[IBIS Ver]   3.2
[File name]   sprm349a.ibs
[File Rev]   1.0
[Date]   Monday Aug 10  2009
[Source]   IBIS Model Generated from PACED 4.51D
[Notes]
|   Technology type SR50
|   Warnings such as non-montonic behavior at the noisy end
|   points of the slopes or TVCurves not asymptotically
|   approaching a final value can be ignored.
[Disclaimer]   Please be aware that in the absence of a written agreement
|   Texas Instruments(TI) assumes no liability for:
|   (1) The accuracy of the IBIS models provided to your company
|   (2) The proper functioning of these Models in your design
|   or for any resulting applications;or
|   property rights resulting from your use of these models.
|   This information is for modeling purposes only
|   and is not guaranteed.
|   TI provides IBIS Models as a service to our customers and
|   therefore reserves the right to limit distribution of the
|   Models.
[Copyright]   Property of Texas Instruments Incorporated.
|   Unauthorised reproduction and/or distribution is strictly.
|   prohibited.
|   This product is protected under copyright law and trade
|   secret law as an unpublished work.
|   Created 1999,(C) Copyright 1999-2001,
|   Texas Instruments Incorporated., All Rights Reserved.
[Component]   C6452   | 529 pin
[Manufacturer]   Texas Instruments
[Package]
| Variable   Typ   Min   Max
R_pkg   0.0   0.0   0.0
L_pkg   0.0   0.0   0.0
C_pkg   0.0   0.0   0.0
[Pin]   signal_name   model_name   R_pin   L_pin   C_pin
M1   CLKIN1   THYPDFZP18   1.03E+00   2.43E-09   1.57E-12
F1   CLKIN2   THYPDFZP18   1.24E+00   3.00E-09   1.65E-12
M3   SYSCLK4   EPUFZSCP18   6.07E-01   2.05E-09   1.32E-12
| JTAG
H23   TCLK   KP18PUSR50   1.14E+00   2.78E-09   1.62E-12
J22   TDI   THYPUFZP18   1.10E+00   2.58E-09   1.66E-12
J23   TDO   EPUFZSCP18   1.16E+00   2.67E-09   1.47E-12
L22   TMS   THYPUFZP18   9.03E-01   2.34E-09   1.52E-12
L23   TRSTz   THYPDFZP18   1.03E+00   2.62E-09   1.41E-12
K23   EMU0   EPUFZSCP18   1.08E+00   2.62E-09   1.49E-12
K22   EMU1   EPUFZSCP18   1.02E+00   2.47E-09   1.58E-12
K21   EMU2   EPUFZSCP18   7.51E-01   2.07E-09   1.39E-12
K20   EMU3   EPUFZSCP18   5.34E-01   1.66E-09   1.26E-12
L18   EMU4   EPUFZSCP18   2.72E-01   1.21E-09   1.07E-12
J21   EMU5   EPUFZSCP18   8.00E-01   2.22E-09   1.48E-12
K19   EMU6   EPUFZSCP18   4.11E-01   1.49E-09   1.19E-12
H21   EMU7   EPUFZSCP18   9.35E-01   2.47E-09   1.51E-12
J20   EMU8   EPUFZSCP18   6.07E-01   1.77E-09   1.33E-12
H20   EMU9   EPUFZSCP18   6.51E-01   1.98E-09   1.35E-12
J19   EMU10   EPUFZSCP18   4.39E-01   1.54E-09   1.18E-12
K18   EMU11   EPUFZSCP18   1.61E-01   1.32E-09   9.70E-13
| Reset/Interrupts
J18   NMI   SHYPDFZP18   1.68E-01   9.30E-10  9.90E-13
H19   RESETSTATz   CSHYPUFZP18   4.23E-01   1.44E-09  1.19E-12
G20   RESETz   IT33SHYP18   7.57E-01   2.04E-09  1.41E-12
|HOST-PORT INTERFACE (HPI) or PCI
AA22   AD00/HD00   CGPDFZP18   1.13E+00   3.06E-09  1.65E-12
AB22   AD01/HD01   CGPDFZP18   1.30E+00   2.94E-09  1.77E-12
AC21   AD02/HD02   CGPDFZP18   1.43E+00   3.03E-09  1.82E-12
AA23   AD03/HD03   CGPDFZP18   1.33E+00   3.36E-09  1.62E-12
AC22   AD04/HD04   CGPDFZP18   1.48E+00   3.26E-09  1.78E-12
AB21   AD05/HD05   CGPDFZP18   1.20E+00   2.86E-09  1.78E-12
AA21   AD06/HD06   CGPDFZP18   1.21E+00   2.84E-09  1.75E-12
Y21   AD07/HD07   CGPDFZP18   9.64E-01   2.45E-09  1.56E-12
AB20   AD08/HD08   CGPDFZP18   1.32E+00   3.07E-09  1.77E-12
AA20   AD09/HD09   CGPDFZP18   1.12E+00   2.60E-09  1.71E-12
Y20   AD10/HD10   CGPDFZP18   9.03E-01   2.30E-09  1.53E-12
Y19   AD11/HD11   CGPDFZP18   7.65E-01   2.00E-09  1.46E-12
AB18   AD12/HD12   CGPDFZP18   1.03E+00   2.44E-09  1.57E-12
AA19   AD13/HD13   CGPDFZP18   9.67E-01   2.55E-09  1.60E-12
AC18   AD14/HD14   CGPDFZP18   1.25E+00   2.84E-09  1.66E-12
AA18   AD15/HD15   CGPDFZP18   9.00E-01   2.41E-09  1.56E-12
Y16   AD16/HD16   CGPDFZP18   5.39E-01   1.78E-09  1.28E-12
AB15   AD17/HD17   CGPDFZP18   8.91E-01   2.20E-09  1.44E-12
AA15   AD18/HD18   CGPDFZP18   6.70E-01   1.96E-09  1.40E-12
Y15   AD19/HD19   CGPDFZP18   5.61E-01   1.77E-09  1.30E-12
W15   AD20/HD20   CGPDFZP18   3.46E-01   1.54E-09  1.13E-12
V15   AD21/HD21   CGPDFZP18   3.24E-01   1.93E-09  1.13E-12
AC14   AD22/HD22   CGPDFZP18   9.71E-01   2.39E-09  1.40E-12
AB14   AD23/HD23   CGPDFZP18   8.86E-01   2.29E-09  1.52E-12
W14   AD24/HD24   CGPDFZP18   2.58E-01   1.37E-09  1.09E-12
V14   AD25/HD25   CGPDFZP18   2.33E-01   1.28E-09  1.03E-12
AC13   AD26/HD26   CGPDFZP18   9.46E-01   2.52E-09  1.41E-12
AB13   AD27/HD27   CGPDFZP18   7.59E-01   2.10E-09  1.23E-12
AA13   AD28/HD28   CGPDFZP18   6.92E-01   2.01E-09  1.37E-12
Y13   AD29/HD29   CGPDFZP18   4.89E-01   1.66E-09  1.24E-12
W13   AD30/HD30   CGPDFZP18   3.65E-01   1.49E-09  1.13E-12
V13   AD31/HD31   CGPDFZP18   1.74E-01   1.14E-09  9.80E-13
W19   PPAR/HASz   CGPUFZP18   7.38E-01   2.23E-09  1.44E-12
Y18   PSTOPz/HCNTL0   CGPDFZP18   7.33E-01   2.05E-09  1.38E-12
Y17   PDEVSELz/HCNTL1   CGPDFZP18   6.59E-01   1.94E-09  1.35E-12
W17   PPERRz/HCSz   CGPUFZP18   5.02E-01   1.71E-09  1.25E-12
W18   PSERRz/HDS1z   CGPUFZP18   5.99E-01   1.94E-09  1.34E-12
AC17   PCBE1z/HDS2z   CGPUFZP18   1.37E+00   3.05E-09  1.74E-12
W16   PCBE2z/HRWz   CGPUFZP18   3.90E-01   1.62E-09  1.18E-12
AC15   PCLK/HHWIL   CGPUFZP18   1.21E+00   2.83E-09  1.65E-12
AA16   PFRAMEz/HINTz   CGPUFZP18   8.21E-01   2.15E-09  1.48E-12
AB17   PIRDYz/HRDYz   CGPUFZP18   8.74E-01   2.33E-09  1.51E-12
U13   PGNTz/GP00   CGPDFZP18   8.20E-02   6.60E-10  9.90E-13
U12   PRSTz/GP01   CGPDFZP18   1.95E-01   1.77E-09  9.90E-13
V12   PINTAz/GP02   CGPDFZP18   1.12E-01   7.50E-10  9.30E-13
AA12   PREQz/GP03   CGPDFZP18   6.04E-01   2.11E-09  1.30E-12
AC20   PCBE0z/GP04   CGPDFZP18   1.50E+00   3.44E-09  1.79E-12
AA17   PTRDYz/GP05   CGPDFZP18   7.78E-01   2.20E-09  1.44E-12
AA14   PIDSEL/GP06   CGPDFZP18   7.10E-01   2.03E-09  1.31E-12
Y14   PCBE3z/GP07   CGPDFZP18   5.13E-01   1.76E-09  1.26E-12
| CONFIGURATION AND EMIFA
F2   DEVICEENABLE0/AEA20 PDFZSCP18   1.10E-03   2.71E-09  1.69E-12
G3   EMIFAWIDTH/AEA22   PDFZSCP18   9.26E-01   2.45E-09  1.55E-12
G2   FASTBOOT/AEA21   PDFZSCP18   9.83E-01   2.39E-09  1.49E-12
H2   UHPIEN   THYPDFZP18   9.16E-01   2.19E-09  1.46E-12
H3   HPIWIDTH/AEA16   PDFZSCP18   6.86E-01   1.84E-09  1.39E-12
H6   RSVBOOT/AEA15   DPUFZSCP18   3.83E-01   1.80E-09  1.17E-12
G5   PCI66/AEA18   PDFZSCP18   6.50E-01   1.95E-09  1.43E-12
F3   BOOTMODE0/AEA11   PDFZSCP18   9.09E-01   2.46E-09  1.57E-12
F4   BOOTMODE1/AEA12   PDFZSCP18   8.43E-01   2.38E-09  1.53E-12
F5   BOOTMODE2/AEA13   PDFZSCP18   7.20E-01   2.13E-09  1.45E-12
G6   BOOTMODE3/AEA14   PDFZSCP18   4.32E-01   1.86E-09  1.30E-12
|I2C
D22   SCL0   BI2CSFZP18   1.07E+00   2.64E-09  1.65E-12
C23   SDA0   BI2CSFZP18   1.34E+00   3.18E-09  1.72E-12
| MDIO
U9   MDCLK   BTHYPDFZP18   4.31E-02   1.01E-09  8.90E-13
U8   MDIO   BTHYPUFZP18   3.15E-01   1.51E-09  1.08E-12
| SPI or UART
F22   SPICLK   CSHYPUFZP18   9.92E-01   2.41E-09  1.5E-12
D23   SPICS1z/UARTTX   CSHYPUFZP18   1.17E+00   2.88E-09  1.63E-12
F23   SPICS2z/UARTRX   CSHYPUFZP18   1.11E+00   2.71E-09  1.47E-12
G23   SPIDI/UARTRTS   CSHYPUFZP18   1.09E+00   2.68E-09  1.36E-12
F21   SPIDO/UARTCTS   CSHYPUFZP18   8.04E-01   2.27E-09  1.48E-12
| TIMER 0/1 or GPIO[8:11]
E20   T0INP12/GP08   CSHYPDFZP18   6.60E-01   1.98E-09  1.36E-12
D21   T0OUT12/GP09   CSHYPDFZP18   8.34E-01   2.18E-09  1.52E-12
E21   T1INP12/GP10   CSHYPDFZP18   7.81E-01   2.11E-09  1.47E-12
C22   T1OUT12/GP11   CSHYPDFZP18   1.13E+00   2.53E-09  1.64E-12
| MCASP
AC4   AHCLKR_TSIP1CLKA   HYPDFZP18   1.27E+00   3.13E-09  1.70E-12
AC3   AHCLKX_TSIP1CLKB   HYPDFZP18   1.37E+00   3.11E-09  1.76E-12
AC6   ACLKR_TSIP0CLKA   PDFZSCP18   1.22E+00   3.03E-09  1.58E-12
AC7   ACLKX_TSIP0CLKB   PDFZSCP18   1.06E+00   2.81E-09  1.59E-12
W6   AFSR_TSIP0FSA   HYPDFZP18   4.85E-01   1.75E-09  1.24E-12
AA7   AFSX_TSIP0FSB   HYPDFZP18   7.10E-01   2.09E-09  1.40E-12
AB6   AXR0_TSIP0TR0   HYPDFZP18   9.44E-01   2.37E-09  1.54E-12
Y6   AXR1_TSIP0TR1   HYPDFZP18   6.21E-01   2.01E-09  1.34E-12
AA6   AXR2_TSIP0TX0   HYPDFZP18   9.61E-01   2.55E-09  1.57E-12
AB4   AXR3_TSIP0TX1   HYPDFZP18   1.10E+00   2.75E-09  1.69E-12
Y5   AXR4_TSIP1TR0   HYPDFZP18   7.78E-01   2.33E-09  1.45E-12
V7   AXR5_TSIP1TR1   HYPDFZP18   2.85E-01   1.44E-09  1.09E-12
AA4   AXR6_TSIP1TX0   HYPDFZP18   8.69E-01   2.37E-09  1.53E-12
V6   AXR7_TSIP1TX1   HYPDFZP18   3.46E-01   1.47E-09  1.11E-12
Y7   AXR8   HYPDFZP18   5.14E-01   1.78E-09  1.26E-12
AA5   AXR9   HYPDFZP18   8.91E-01   2.30E-09  1.53E-12
AB3   AMUTEIN_TSIP1FSA   HYPDFZP18   1.08E+00   2.69E-09  1.62E-12
U7   AMUTE_TSIP1FSB   HYPDFZP18   9.10E-02   1.07E-09  9.00E-13
|GPIO[12:15]
V21   GP12   PDFZSCP18   7.68E-01   2.09E-09  1.39E-12
T19   GP13   PDFZSCP18   2.80E-01   1.46E-09  1.09E-12
T20   GP14   PDFZSCP18   5.40E-01   1.81E-09  1.29E-12
T21   GP15   PDFZSCP18   6.41E-01   1.96E-09  1.34E-12
|GPIO[16:31]
R19   GP16   PDFZSCP18   3.50E-01   1.59E-09  1.12E-12
P19   GP17   PDFZSCP18   2.74E-01   1.37E-09  1.08E-12
P18   GP18   PDFZSCP18   5.46E-02   8.00E-10  9.20E-13
R22   GP19   PDFZSCP18   7.90E-01   2.27E-09  1.39E-12
R21   GP20   PDFZSCP18   6.22E-01   1.90E-09  1.18E-12
R20   GP21   PDFZSCP18   4.22E-01   1.59E-09  1.19E-12
N21   GP22   PDFZSCP18   6.84E-01   1.87E-09  1.34E-12
N20   GP23   PDFZSCP18   4.77E-01   1.60E-09  1.23E-12
N19   GP24   PDFZSCP18   3.36E-01   1.45E-09  1.12E-12
P21   GP25   PDFZSCP18   6.15E-01   1.78E-09  1.32E-12
P20   GP26   PDFZSCP18   4.98E-01   1.67E-09  1.23E-12
M20   GP27   PDFZSCP18   4.31E-01   1.55E-09  1.20E-12
M18   GP28   PDFZSCP18   2.42E-01   9.50E-10  1.05E-12
N18   GP29   PDFZSCP18   1.11E-01   1.36E-09  9.30E-13
M21   GP30   PDFZSCP18   6.50E-01   1.91E-09  1.37E-12
M19   GP31   PDFZSCP18   3.69E-01   1.50E-09  1.16E-12
|VLYNQ
W1   VCLK   EPUFZSCP18   1.37E+00   2.98E-09  1.82E-12
Y1   VSCRUNz   DPUFZSCP18   1.21E+00   2.87E-09  1.56E-12
W2   VRXD0   PDFZSCP18   1.04E+00   2.57E-09  1.57E-12
V3   VRXD1   PDFZSCP18   7.50E-01   2.13E-09  1.43E-12
V4   VRXD2   PDFZSCP18   6.91E-01   1.93E-09  1.37E-12
U1   VRXD3   PDFZSCP18   1.11E+00   2.71E-09  1.39E-12
U3   VTXD0   PDFZSCP18   6.30E-01   2.07E-09  1.36E-12
U2   VTXD1   PDFZSCP18   9.93E-01   2.48E-09  1.55E-12
U5   VTXD2   PDFZSCP18   4.26E-01   1.65E-09  1.18E-12
U4   VTXD3   PDFZSCP18   5.54E-01   1.83E-09  1.28E-12
|EMIFA
T1   AECLKIN   PDFZSCP18   1.10E+00   2.68E-09  1.57E-12
P1   AECLKOUT   ETHYPDFZSCP18   1.29E+00   3.05E-09  1.58E-12
T2   ASDWEz   DPUFZSCP18   9.53E-01   2.50E-09  1.48E-12
R1   ARNW   DPUFZSCP18   1.16E+00   2.90E-09  1.56E-12
P2   AOE   DPUFZSCP18   1.35E+00   3.01E-09  1.88E-12
T6   AED00   DPUFZSCP18   4.61E-01   1.80E-09  1.23E-12
T5   AED01   DPUFZSCP18   4.48E-01   1.70E-09  1.20E-12
T4   AED02   DPUFZSCP18   5.57E-01   1.94E-09  1.29E-12
T3   AED03   DPUFZSCP18   6.26E-01   2.10E-09  1.36E-12
R6   AED04   DPUFZSCP18   2.37E-01   1.30E-09  1.05E-12
R5   AED05   DPUFZSCP18   3.55E-01   1.68E-09  1.13E-12
R4   AED06   DPUFZSCP18   6.30E-01   1.99E-09  1.34E-12
R3   AED07   DPUFZSCP18   7.59E-01   2.16E-09  1.44E-12
R2   AED08   DPUFZSCP18   7.50E-01   2.10E-09  1.47E-12
P6   AED09   DPUFZSCP18   1.95E-01   1.17E-09  1.00E-12
P5   AED10   DPUFZSCP18   2.95E-01   1.57E-09  1.10E-12
P4   AED11   DPUFZSCP18   4.27E-01   1.71E-09  1.19E-12
P3   AED12   DPUFZSCP18   6.58E-01   2.05E-09  1.39E-12
N4   AED13   DPUFZSCP18   4.47E-01   1.74E-09  1.20E-12
N6   AED14   DPUFZSCP18   1.75E-01   1.02E-09  9.60E-13
N5   AED15   DPUFZSCP18   2.68E-01   1.44E-09  1.05E-12
|EMIFA
L1   AARDY   DPUFZSCP18   1.28E+00   3.17E-09  1.67E-12
J2   ABA0   PDFZSCP18   1.04E+00   2.46E-09  1.59E-12
J1   ABA1   PDFZSCP18   1.45E+00   3.33E-09  1.81E-12
K2   AADS   PDFZSCP18   1.04E+00   2.68E-09  1.62E-12
L2   ABE00z   DPUFZSCP18   8.08E-01   2.14E-09  1.47E-12
M4   ABE01z   DPUFZSCP18   4.85E-01   2.09E-09  1.24E-12
M5   AEA10   DPUFZSCP18   2.77E-01   1.46E-09  1.10E-12
L3   ACE2z   DPUFZSCP18   6.73E-01   2.12E-09  1.37E-12
L4   ACE3z   DPUFZSCP18   4.76E-01   1.85E-09  1.21E-12
L5   AEA00   PDFZSCP18   3.66E-01   1.74E-09  1.15E-12
K3   AEA01   PDFZSCP18   8.15E-01   2.25E-09  1.44E-12
K4   AEA02   PDFZSCP18   5.73E-01   1.83E-09  1.30E-12
L6   AEA03   PDFZSCP18   2.93E-01   1.53E-09  1.11E-12
K5   AEA04   PDFZSCP18   4.35E-01   1.59E-09  1.22E-12
J3   AEA05   PDFZSCP18   7.12E-01   2.06E-09  1.42E-12
J4   AEA06   PDFZSCP18   6.99E-01   2.11E-09  1.39E-12
J5   AEA07   PDFZSCP18   5.03E-01   1.86E-09  1.26E-12
J6   AEA08   PDFZSCP18   4.17E-01   1.44E-09  1.22E-12
K6   AEA09   PDFZSCP18   2.68E-01   1.39E-09  1.08E-12
|EMIFA
H4   AEA23   PDFZSCP18   6.03E-01   1.81E-09  1.33E-12
H5   AEA19   DPUFZSCP18   4.13E-01   1.63E-09  1.24E-12
G4   AECLKINSEL/AEA17   PDFZSCP18   7.59E-01   2.14E-09  1.45E-12
|DDR2 Memory Controller
C12   DDR_BA0   BSSTL18GFZ   7.13E-01   2.24E-09  1.37E-12
B12   DDR_BA1   BSSTL18GFZ   9.90E-01   2.87E-09  1.57E-12
E11   DDR_BA2   BSSTL18GFZ   3.69E-01   1.57E-09  1.13E-12
F9   DDR_CSz   BSSTL18GFZ   1.55E-01   9.90E-10  1.00E-12
D15   DDR_A00   BSSTL18GFZ   7.89E-01   2.19E-09  1.45E-12
C15   DDR_A01   BSSTL18GFZ   8.92E-01   2.34E-09  1.53E-12
F13   DDR_A02   BSSTL18GFZ   3.48E-01   1.56E-09  1.20E-12
E14   DDR_A03   BSSTL18GFZ   5.23E-01   1.84E-09  1.29E-12
D14   DDR_A04   BSSTL18GFZ   6.56E-01   2.26E-09  1.35E-12
C14   DDR_A05   BSSTL18GFZ   8.44E-01   2.42E-09  1.49E-12
F11   DDR_A06   BSSTL18GFZ   1.97E-01   1.14E-09  1.00E-12
B14   DDR_A07   BSSTL18GFZ   9.61E-01   2.66E-09  1.45E-12
F12   DDR_A08   BSSTL18GFZ   3.14E-01   1.58E-09  1.16E-12
D13   DDR_A09   BSSTL18GFZ   5.99E-01   2.06E-09  1.32E-12
A13   DDR_A10   BSSTL18GFZ   1.07E+00   2.70E-09  1.58E-12
B13   DDR_A11   BSSTL18GFZ   9.79E-01   2.58E-09  1.50E-12
E12   DDR_A12   BSSTL18GFZ   4.73E-01   1.78E-09  1.22E-12
F10   DDR_A13   BSSTL18GFZ   2.59E-01   1.34E-09  1.11E-12
A12   DDR_CLKN   BSSTL18GFZ   1.07E+00   2.61E-09  1.54E-12
A11   DDR_CLKP   BSSTL18GFZ   1.06E+00   2.52E-09  1.51E-12
E9   DDR_D00   BSSTL18GFZ   2.79E-01   1.37E-09  1.08E-12
C9   DDR_D01   BSSTL18GFZ   7.42E-01   2.03E-09  1.41E-12
B9   DDR_D02   BSSTL18GFZ   8.01E-01   2.33E-09  1.37E-12
C8   DDR_D03   BSSTL18GFZ   6.80E-01   2.06E-09  1.35E-12
E8   DDR_D04   BSSTL18GFZ   2.66E-01   1.23E-09  1.06E-12
D8   DDR_D05   BSSTL18GFZ   5.70E-01   1.82E-09  1.31E-12
C7   DDR_D06   BSSTL18GFZ   6.64E-01   1.96E-09  1.30E-12
E7   DDR_D07   BSSTL18GFZ   3.81E-01   1.51E-09  1.17E-12
C6   DDR_D08   BSSTL18GFZ   7.33E-01   2.12E-09  1.40E-12
B7   DDR_D09   BSSTL18GFZ   8.07E-01   2.19E-09  1.45E-12
D6   DDR_D10   BSSTL18GFZ   6.12E-01   1.98E-09  1.32E-12
A3   DDR_D11   BSSTL18GFZ   1.30E+00   3.23E-09  1.59E-12
B3   DDR_D12   BSSTL18GFZ   1.18E+00   2.81E-09  1.65E-12
A4   DDR_D13   BSSTL18GFZ   1.06E+00   2.72E-09  1.60E-12
B4   DDR_D14   BSSTL18GFZ   9.80E-01   2.53E-09  1.51E-12
C5   DDR_D15   BSSTL18GFZ   7.44E-01   2.27E-09  1.42E-12
B16   DDR_D16   BSSTL18GFZ   1.14E+00   2.74E-09  1.60E-12
C16   DDR_D17   BSSTL18GFZ   1.03E+00   2.67E-09  1.61E-12
D16   DDR_D18   BSSTL18GFZ   8.61E-01   2.33E-09  1.46E-12
E16   DDR_D19   BSSTL18GFZ   7.90E-01   2.29E-09  1.38E-12
B17   DDR_D20   BSSTL18GFZ   1.20E+00   2.84E-09  1.71E-12
C17   DDR_D21   BSSTL18GFZ   1.11E+00   2.73E-09  1.38E-12
D17   DDR_D22   BSSTL18GFZ   9.15E-01   2.28E-09  1.42E-12
E17   DDR_D23   BSSTL18GFZ   8.53E-01   2.19E-09  1.49E-12
C18   DDR_D24   BSSTL18GFZ   1.26E+00   3.10E-09  1.75E-12
D18   DDR_D25   BSSTL18GFZ   1.06E+00   2.53E-09  1.50E-12
B19   DDR_D26   BSSTL18GFZ   1.50E+00   3.33E-09  1.82E-12
C19   DDR_D27   BSSTL18GFZ   1.28E+00   3.03E-09  1.73E-12
B20   DDR_D28   BSSTL18GFZ   1.47E+00   3.34E-09  1.86E-12
D19   DDR_D29   BSSTL18GFZ   1.07E+00   2.59E-09  1.54E-12
C20   DDR_D30   BSSTL18GFZ   1.35E+00   2.98E-09  1.86E-12
E19   DDR_D31   BSSTL18GFZ   9.30E-01   2.44E-09  1.41E-12
E13   DDR_ODT0   BSSTL18GFZ   5.03E-01   1.80E-09  1.22E-12
A14   DDR_ODT1   BSSTL18GFZ   1.12E+00   2.86E-09  1.52E-12
D10   DDR_CASz   BSSTL18GFZ   5.47E-01   1.81E-09  1.28E-12
B11   DDR_CKE   BSSTL18GFZ   8.13E-01   2.31E-09  1.46E-12
D7   DDR_DQGATE0   BSSTL18GFZ   4.51E-01   1.52E-09  1.22E-12
B6   DDR_DQGATE1   BSSTL18GFZ   8.65E-01   2.22E-09  1.36E-12
E18   DDR_DQGATE2   BSSTL18GFZ   9.05E-01   2.25E-09  1.48E-12
A21   DDR_DQGATE3   BSSTL18GFZ   1.92E+00   4.16E-09  2.25E-12
B8   DDR_DQM0   BSSTL18GFZ   7.38E-01   2.05E-09  1.35E-12
D5   DDR_DQM1   BSSTL18GFZ   6.96E-01   2.18E-09  1.38E-12
E15   DDR_DQM2   BSSTL18GFZ   6.82E-01   2.08E-09  1.36E-12
B21   DDR_DQM3   BSSTL18GFZ   1.70E+00   3.54E-09  2.15E-12
A9   DDR_DQS0P   BSSTL18GFZ   1.32E+00   2.99E-09  1.69E-12
A7   DDR_DQS1P   BSSTL18GFZ   1.20E+00   2.80E-09  1.65E-12
A17   DDR_DQS2P   BSSTL18GFZ   1.49E+00   3.40E-09  1.72E-12
A20   DDR_DQS3P   BSSTL18GFZ   1.70E+00   3.49E-09  1.85E-12
A8   DDR_DQS0N   BSSTL18GFZ   1.32E+00   2.83E-09  1.66E-12
A6   DDR_DQS1N   BSSTL18GFZ   1.20E+00   2.77E-09  1.57E-12
A16   DDR_DQS2N   BSSTL18GFZ   1.48E+00   3.08E-09  1.87E-12
A19   DDR_DQS3N   BSSTL18GFZ   1.70E+00   3.53E-09  2.04E-12
E10   DDR_RASz   BSSTL18GFZ   3.55E-01   1.53E-09  1.13E-12
D11   DDR_WEz   BSSTL18GFZ   6.52E-01   2.10E-09  1.33E-12
| Reserved Pins
|L20   RSV 1
|L21   RSV 2
|D2   RSV 3
|D1   RSV 4
|D4   RSV 5
|D3   RSV 6
|H7   RSV 7
|H8   RSV 8
|M2   RSV 9
|A2   RSV 10
|E2   RSV 11
|E1   RSV 12
|E4   RSV 13
|E3   RSV 14
|A10   RSV 15
|A22   RSV 16
|V10   RSV 17
|F6   RSV 18
|C2   RSV 19
|C1   RSV 20
|Y12   RSV 21
|W12   RSV 22
|   Component BI2CSFZP18 -Aug 18, 2006 Rev 1.0
[Model Selector] BI2CSFZP18
BI2CSFZP18_COM_3P3  Cell operated at 3.3(nom) COM TEMP MODE
BI2CSFZP18_IND_3P3  Cell operated at 3.3(nom) IND TEMP MODE
|   Component BPCI66RCGPDFZP18 -Aug 22, 2006 Rev 1.0
|   Shortened Model Name is  CGPDFZP18
[Model Selector] CGPDFZP18
CGPDFZP18_M2_COM_3P3  Cell operated at 3.3(nom) COM TEMP MODE2
|BUFFER OPERATING AT 100UA WITH PULLDOWN ON AT COM TEMP
CGPDFZP18_M1_COM_3P3  Cell operated at 3.3(nom) COM TEMP MODE1
|BUFFER OPERATING IN NORMAL MODE AT COM TEMP
CGPDFZP18_M2_IND_3P3  Cell operated at 3.3(nom) IND TEMP MODE2
|BUFFER OPERATING AT 100UA WITH PULLDOWN ON AT IND TEMP
CGPDFZP18_M1_IND_3P3  Cell operated at 3.3(nom) IND TEMP MODE1
|   Component BPCI66RCGPUFZP18 -Aug 22, 2006 Rev 1.0
|   Shortened Model Name is CGPUFZP18
[Model Selector] CGPUFZP18
CGPUFZP18_M2_COM_3P3  Cell operated at 3.3(nom) COM TEMP MODE2
|BUFFER OPERATING AT 100UA WITH PULLUP ON AT COM TEMP
CGPUFZP18_M1_COM_3P3  Cell operated at 3.3(nom) COM TEMP MODE1
|BUFFER OPERATING IN NORMAL MODE AT COM TEMP
CGPUFZP18_M2_IND_3P3  Cell operated at 3.3(nom) IND TEMP MODE2
|BUFFER OPERATING AT 100UA WITH PULLUP ON AT IND TEMP
CGPUFZP18_M1_IND_3P3  Cell operated at 3.3(nom) IND TEMP MODE1
|   Component BT3325ETHYPDFZSCP18 -May 28, 2007 Rev 1.1
|   Shortened Model Name is ETHYPDFZSCP18
[Model Selector] ETHYPDFZSCP18
PU_OFF_COM5_M6_3P3  Cell operated at 3.3(nom)
|PU_OFF_COM5_M6_3P3BUFFER IN SLOWEST MODE WITH COMTEMP AT PLUS OR MINUS 5PE
|RCENT VDDS WITH PULLDOWN OFF
PU_ON_COM5_M3_3P3  Cell operated at 3.3(nom)
|PU_ON_COM5_M3_3P3BUFFER OPERATING AT 100UA IN SLOWEST MODE WITH COMTEMP AT
| PLUS OR MINUS 5PERCENT VDDS WITH PULLDOWN ON
PU_OFF_IND5_M6_3P3  Cell operated at 3.3(nom)
|PU_OFF_IND5_M6_3P3BUFFER IN SLOWEST MODE WITH INDTEMP AT PLUS OR MINUS 5PE
|RCENT VDDS WITH PULLDOWN OFF
PU_ON_IND5_M3_3P3  Cell operated at 3.3(nom)
|   Component BT3325ETHYPUFZSCP18 -May 28, 2007 Rev 1.1
|   Note: Shortened Model name is EPUFZSCP18
[Model Selector] EPUFZSCP18
BPU_OFF_COM5_M6_3P3  Cell operated at 3.3(nom)
|BPU_OFF_COM5_M6_3P3BUFFER IN SLOWEST MODE WITH COMTEMP AT PLUS OR MINUS 5PE
|RCENT VDDS WITH PULLUP OFF
BPU_ON_COM5_M3_3P3  Cell operated at 3.3(nom)
|BPU_ON_COM5_M3_3P3BUFFER OPERATING AT 100UA IN SLOWEST MODE WITH COMTEMP AT
| PLUS OR MINUS 5PERCENT VDDS WITH PULLUP ON
BPU_OFF_IND5_M6_3P3  Cell operated at 3.3(nom)
|BPU_OFF_IND5_M6_3P3BUFFER IN SLOWEST MODE WITH INDTEMP AT PLUS OR MINUS 5PE
|RCENT VDDS WITH PULLUP OFF
BPU_ON_IND5_M3_3P3  Cell operated at 3.3(nom)
|   Component BT3350BTHYPDFZP18
|   Shortened Model Name is BTHYPDFZP18
[Model Selector] BTHYPDFZP18
MODE1_COM5_3P3  Cell operated at 3.3(nom)
|MODE1_COM5_3P3BUFFER OPERATING AT 100UA WITH COMTEMP AT PLUS OR MINUS 5PER
|CENT VDDS WITH PULLDOWN ON
MODE4_COM5_3P3  Cell operated at 3.3(nom)
|MODE4_COM5_3P3BUFFER IN NORMAL MODE WITH COMTEMP AT PLUS OR MINUS 5PERCENT
| VDDS
MODE1_IND5_3P3  Cell operated at 3.3(nom)
|MODE1_IND5_3P3BUFFER OPERATING AT 100UAWITH INDTEMP AT PLUS OR MINUS 5PERC
|ENT VDDS WITH PULLDOWN ON
MODE4_IND5_3P3  Cell operated at 3.3(nom)
|   Component BT3350BTHYPUFZP18 Jan 21, 2007 Rev 1.0
|   Shortened Model Name is BTHYPUFZP18
[Model Selector] BTHYPUFZP18
HYPUFZP18_M2_IND_3P3  Cell operated at 3.3(nom) IND TEMP MODE2
HYPUFZP18_M1_IND_3P3  Cell operated at 3.3(nom) IND TEMP MODE1
HYPUFZP18_M2_COM_3P3  Cell operated at 3.3(nom) COM TEMP MODE2
HYPUFZP18_M1_COM_3P3  Cell operated at 3.3(nom) COM TEMP MODE1
|   Component BT3350CSHYPDFZP18
|   Shortened Model Name is CSHYPDFZP18
[Model Selector] CSHYPDFZP18
AMODE1_COM5_3P3  Cell operated at 3.3(nom)
|AMODE1_COM5_3P3BUFFER OPERATING AT 100UA WITH COMTEMP AT PLUS OR MINUS 5PER
|CENT VDDS WITH PULLDOWN ON
AMODE4_COM5_3P3  Cell operated at 3.3(nom)
|AMODE4_COM5_3P3BUFFER IN NORMAL MODE WITH COMTEMP AT PLUS OR MINUS 5PERCENT
| VDDS
AMODE1_IND5_3P3  Cell operated at 3.3(nom)
|AMODE1_IND5_3P3BUFFER OPERATING AT 100UAWITH INDTEMP AT PLUS OR MINUS 5PERC
|ENT VDDS WITH PULLDOWN ON
AMODE4_IND5_3P3  Cell operated at 3.3(nom)
|   Component BT3350CSHYPUFZP18
|   Shortened Model Name is CSHYPUFZP18
[Model Selector] CSHYPUFZP18
CMODE1_COM5_3P3  Cell operated at 3.3(nom)
|CMODE1_COM5_3P3BUFFER OPERATING AT 100UA WITH COMTEMP AT PLUS OR MINUS 5PER
|CENT VDDS WITH PULLUP ON
CMODE4_COM5_3P3  Cell operated at 3.3(nom)
|CMODE4_COM5_3P3BUFFER OPERATING IN NORMAL MODE WITH COM TEMP AT PLUS OR MIN
|US 5PERCENT VDDS
CMODE1_IND5_3P3  Cell operated at 3.3(nom)
|CMODE1_IND5_3P3BUFFER OPERATING AT 100UA WITH INDTEMP AT PLUS OR MINUS 5PER
|CENT VDDS WITH PULLUP ON
CMODE4_IND5_3P3  Cell operated at 3.3(nom)
|   Component BT3350CTHYPDFZP18
|   Shortened Model Name is HYPDFZP18
[Model Selector] HYPDFZP18
HMODE1_COM5_3P3  Cell operated at 3.3(nom)
|HMODE1_COM5_3P3BUFFER OPERATING AT 100UA WITH COMTEMP AT PLUS OR MINUS 5PER
|CENT VDDS WITH PULLDOWN ON
HMODE4_COM5_3P3  Cell operated at 3.3(nom)
|HMODE4_COM5_3P3BUFFER IN NORMAL MODE WITH COMTEMP AT PLUS OR MINUS 5PERCENT
| VDDS
HMODE1_IND5_3P3  Cell operated at 3.3(nom)
|HMODE1_IND5_3P3BUFFER OPERATING AT 100UAWITH INDTEMP AT PLUS OR MINUS 5PERC
|ENT VDDS WITH PULLDOWN ON
HMODE4_IND5_3P3  Cell operated at 3.3(nom)
|   Component BT3350DTHYPDFZSCP18 May 23, 2007 Rev 1.0
|   Shortened Model Name is PDFZSCP18
[Model Selector] PDFZSCP18
PPU_OFF_COM5_M6_3P3  Cell operated at 3.3(nom)
|PPU_OFF_COM5_M6_3P3BUFFER IN SLOWEST MODE WITH COMTEMP AT PLUS OR MINUS 5PE
|RCENT VDDS WITH PULLDOWN OFF
PPU_ON_COM5_M3_3P3  Cell operated at 3.3(nom)
|PPU_ON_COM5_M3_3P3BUFFER OPERATING AT 100UA IN SLOWEST MODE WITH COMTEMP AT
| PLUS OR MINUS 5PERCENT VDDS WITH PULLDOWN ON
PPU_OFF_IND5_M6_3P3  Cell operated at 3.3(nom)
|PPU_OFF_IND5_M6_3P3BUFFER IN SLOWEST MODE WITH INDTEMP AT PLUS OR MINUS 5PE
|RCENT VDDS WITH PULLDOWN OFF
PPU_ON_IND5_M3_3P3  Cell operated at 3.3(nom)
|   Component BT3350DTHYPUFZSCP18 May 23, 2007 Rev 1.0
|   Shortened Model Name is DPUFZSCP18
[Model Selector] DPUFZSCP18
DPU_OFF_COM5_M6_3P3  Cell operated at 3.3(nom)
|DPU_OFF_COM5_M6_3P3BUFFER IN SLOWEST MODE WITH COMTEMP AT PLUS OR MINUS 5PE
|RCENT VDDS WITH PULLDOWN OFF
DPU_ON_COM5_M3_3P3  Cell operated at 3.3(nom)
|DPU_ON_COM5_M3_3P3BUFFER OPERATING AT 100UA IN SLOWEST MODE WITH COMTEMP AT
| PLUS OR MINUS 5PERCENT VDDS WITH PULLDOWN ON
DPU_OFF_IND5_M6_3P3  Cell operated at 3.3(nom)
|DPU_OFF_IND5_M6_3P3BUFFER IN SLOWEST MODE WITH INDTEMP AT PLUS OR MINUS 5PE
|RCENT VDDS WITH PULLDOWN OFF
DPU_ON_IND5_M3_3P3  Cell operated at 3.3(nom)
|   Component IQ33TTCKP18PUSR50 Jul 31, 2006 Rev 1.0
|   Shortened Model Name is KP18PUSR50
[Model Selector] KP18PUSR50
KP18PUSR50_MODE2_M1  Cell operated at 3.3V & IND temp with Pullup On
KP18PUSR50_MODE1_M1  Cell operated at 3.3V & IND temp with Pullup Off
KP18PUSR50_MODE2_M2  Cell operated at 3.3V & COM temp with Pullup On
KP18PUSR50_MODE1_M2  Cell operated at 3.3V & COM temp with Pullup Off
|   Component IT33SHYP18 Mar 23, 2007 Rev 1.0
[Model Selector] IT33SHYP18
IT33SHYP18_3P3_COM  Cell operated at 3.3(nom)
|IT33SHYP18_3P3BUFFER WITHOUT PULLUP/PULLDOWN
IT33SHYP18_3P3_IND  Cell operated at 3.3(nom)
|IT33SHYP18_3P3BUFFER WITHOUT PULLUP/PULLDOWN
IT33SHYP18_3P3_IN  Cell operated at 3.3(nom)
|IT33SHYP18_3P3BUFFER WITHOUT PULLUP/PULLDOWN
IT33SHYP18_3P3_CM  Cell operated at 3.3(nom)
|   Component IT33SHYPDFZP18 Mar 23, 2007 Rev 1.0
|   Shortened Model Name is SHYPDFZP18
[Model Selector] SHYPDFZP18
SMODE1_COM5_3P3  Cell operated at 3.3(nom)
|SMODE1_COM5_3P3BUFFER OPERATING AT 100UA WITH COMTEMP AT 5PERCENT VDDS WITH
| PULLDOWN ON
SMODE4_COM5_3P3  Cell operated at 3.3(nom)
|SMODE4_COM5_3P3BUFFER IN NORMAL MODE WITH COMTEMP AT 5PERCENT VDDS
SMODE1_IND5_3P3  Cell operated at 3.3(nom)
|SMODE1_IND5_3P3BUFFER OPERATING AT 100UAWITH INDTEMP AT 5PERCENT VDDS WITH
|PULLDOWN ON
SMODE4_IND5_3P3  Cell operated at 3.3(nom)
|   Component IT33THYPDFZP18 Mar 23, 2007 Rev 1.0
|   Note: Shortened model name is THYPDFZP18
[Model Selector] THYPDFZP18
TMODE1_COM5_3P3  Cell operated at 3.3(nom)
|TMODE1_COM5_3P3BUFFER OPERATING AT 100UA WITH COMTEMP AT 5PERCENT VDDS WITH
| PULLDOWN ON
TMODE4_COM5_3P3  Cell operated at 3.3(nom)
|TMODE4_COM5_3P3BUFFER IN NORMAL MODE WITH COMTEMP AT 5PERCENT VDDS
TMODE1_IND5_3P3  Cell operated at 3.3(nom)
|TMODE1_IND5_3P3BUFFER OPERATING AT 100UAWITH INDTEMP AT 5PERCENT VDDS WITH
|PULLDOWN ON
TMODE4_IND5_3P3  Cell operated at 3.3(nom)
|   Component IT33THYPUFZP18 Mar 23, 2007 Rev 1.0
|   Shortened Model Name is THYPUFZP18
[Model Selector] THYPUFZP18
IMODE1_COM5_3P3  Cell operated at 3.3(nom)
|IMODE1_COM5_3P3BUFFER OPERATING AT 100UA WITH COMTEMP AT 5PERCENT VDDS WITH
| PULLUP ON
IMODE4_COM5_3P3  Cell operated at 3.3(nom)
|IMODE4_COM5_3P3BUFFER IN NORMAL MODE WITH COMTEMP AT 5PERCENT VDDS
IMODE1_IND5_3P3  Cell operated at 3.3(nom)
|IMODE1_IND5_3P3BUFFER OPERATING AT 100UAWITH INDTEMP AT 5PERCENT VDDS WITH
|PULLUP ON
IMODE4_IND5_3P3  Cell operated at 3.3(nom)
|   SR50 Cell BSSTL18GFZ
|   Component BSSTL18GFZ
[Component]   BSSTL18GFZ
[Manufacturer]   Texas Instruments
[Package]
| Variable   Typ   Min   Max
R_pkg   0.0   0.0   0.0
L_pkg   0.0   0.0   0.0
C_pkg   0.0   0.0   0.0
[Pin]   signal_name   model_name   R_pin   L_pin   C_pin
VDDS   VDDS   POWER
PAD   PAD   BSSTL18GFZ
VSS   VSS   GND
[Model Selector] BSSTL18GFZ
|FULL TERMINATION WHEN HALFTERM=0 AND ENTERM =1
|HALF TERMINATION WHEN HALFTERM=1 AND ENTERM=1
|NO TERMINATION WHEN HALFTERM=ENTERM=0
|HALFTERM IS HALF STRENGTH THEVININ TERMINATION
|FULLTERM IS FULL STRENGTH THEVININ TERMINATION
|ENTERM MEANS ENABLE THEVENIN TERMINATION
|SR0 AND SR1 ARE SLEW RATE CONTROL PINS.
SR00_NOTERM_IND_1P8  Cell operated at 1.8(nom) FASTEST MODE SR0=SR1=0 IND TEMP
|BUFFER OPERATES IN FASTEST MODE AT IND TEMP WHEN SR0=SR1=0
SR00_NOTERM_COM_1P8  Cell operated at 1.8(nom) FASTEST MODE SR0=SR1=0 COM TEMP
| Models and submodels in the file (68): BI2CSFZP18_COM_3P3 (I/O_open_drain), BI2CSFZP18_IND_3P3 (I/O_open_drain), CGPDFZP18_M2_COM_3P3 (I/O), CGPDFZP18_M1_COM_3P3 (I/O), CGPDFZP18_M2_IND_3P3 (I/O), CGPDFZP18_M1_IND_3P3 (I/O), CGPUFZP18_M2_COM_3P3 (I/O), CGPUFZP18_M1_COM_3P3 (I/O), CGPUFZP18_M2_IND_3P3 (I/O), CGPUFZP18_M1_IND_3P3 (I/O), PU_OFF_COM5_M6_3P3 (I/O), PU_ON_COM5_M3_3P3 (I/O), PU_OFF_IND5_M6_3P3 (I/O), PU_ON_IND5_M3_3P3 (I/O), BPU_OFF_COM5_M6_3P3 (I/O), BPU_ON_COM5_M3_3P3 (I/O), BPU_OFF_IND5_M6_3P3 (I/O), BPU_ON_IND5_M3_3P3 (I/O), MODE1_COM5_3P3 (I/O), MODE4_COM5_3P3 (I/O), MODE1_IND5_3P3 (I/O), MODE4_IND5_3P3 (I/O), HYPUFZP18_M2_IND_3P3 (I/O), HYPUFZP18_M1_IND_3P3 (I/O), HYPUFZP18_M2_COM_3P3 (I/O), HYPUFZP18_M1_COM_3P3 (I/O), AMODE1_COM5_3P3 (I/O), AMODE4_COM5_3P3 (I/O), AMODE1_IND5_3P3 (I/O), AMODE4_IND5_3P3 (I/O), CMODE1_COM5_3P3 (I/O), CMODE4_COM5_3P3 (I/O), CMODE1_IND5_3P3 (I/O), CMODE4_IND5_3P3 (I/O), HMODE1_COM5_3P3 (I/O), HMODE4_COM5_3P3 (I/O), HMODE1_IND5_3P3 (I/O), HMODE4_IND5_3P3 (I/O), PPU_OFF_COM5_M6_3P3 (I/O), PPU_ON_COM5_M3_3P3 (I/O), PPU_OFF_IND5_M6_3P3 (I/O), PPU_ON_IND5_M3_3P3 (I/O), DPU_OFF_COM5_M6_3P3 (I/O), DPU_ON_COM5_M3_3P3 (I/O), DPU_OFF_IND5_M6_3P3 (I/O), DPU_ON_IND5_M3_3P3 (I/O), KP18PUSR50_MODE2_M1 (Input), KP18PUSR50_MODE1_M1 (Input), KP18PUSR50_MODE2_M2 (Input), KP18PUSR50_MODE1_M2 (Input), IT33SHYP18_3P3_COM (Input), IT33SHYP18_3P3_IND (Input), IT33SHYP18_3P3_IN (Input), IT33SHYP18_3P3_CM (Input), SMODE1_COM5_3P3 (Input), SMODE4_COM5_3P3 (Input), SMODE1_IND5_3P3 (Input), SMODE4_IND5_3P3 (Input), TMODE1_COM5_3P3 (Input), TMODE4_COM5_3P3 (Input), TMODE1_IND5_3P3 (Input), TMODE4_IND5_3P3 (Input), IMODE1_COM5_3P3 (Input), IMODE4_COM5_3P3 (Input), IMODE1_IND5_3P3 (Input), IMODE4_IND5_3P3 (Input), SR00_NOTERM_IND_1P8 (3-state), SR00_NOTERM_COM_1P8 (3-state)
